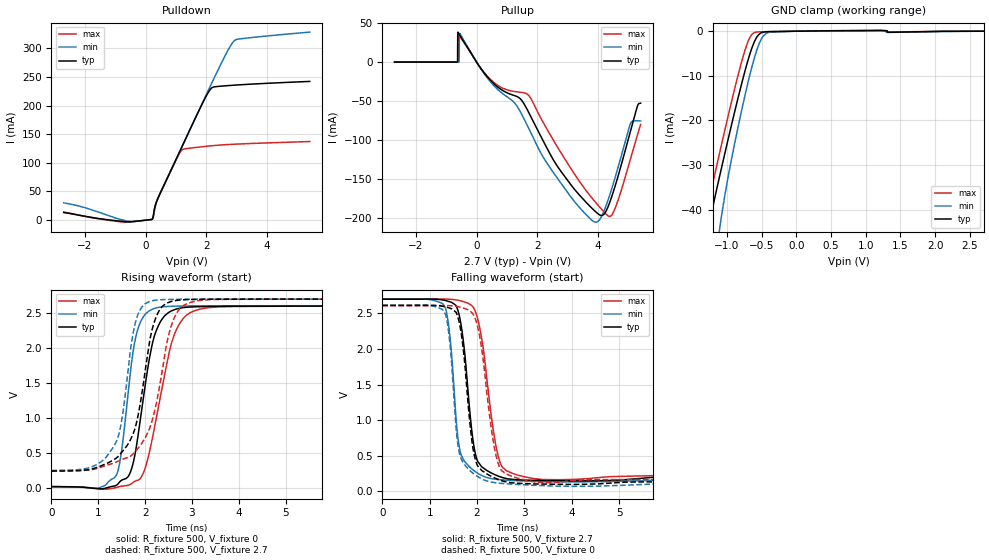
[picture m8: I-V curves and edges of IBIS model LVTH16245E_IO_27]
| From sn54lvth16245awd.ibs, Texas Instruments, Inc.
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[Model]   LVTH16245E_IO_27
Model_type  I/O
Vinl=0.945
Vinh=1.75
Enable   Active-Low
Vref =   0
Rref =   500
Cref =   50p
Vmeas =   1.5
| variable   typ   min   max
C_comp   3.31pF   2.51pF   4.02pF
| C_pullup   5.53pF   0.96pF   13.97pF
| C_pulldown   3.35pF   2.55pF   4.14pF
| C_tri-state   3.31pF   2.51pF   4.02pF
[Temperature Range]   40   100   -40
| Ambient temperature   25   85   -40
[Voltage range]   2.7   2.7   2.7
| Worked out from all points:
|   slope of the pulldown table from 0 to 0.405 V, typ, clamps not added: 10.5 ohm
|   slope of the pullup table from 0 to 0.405 V, typ, clamps not added: 19.2 ohm
|   GND clamp passes 1 mA (typ) near -0.55 V on its own axis
|   rising waveform, R_fixture 500, V_fixture 0: 20-80 % time 364ps typ, 280ps min, 471ps max; typ from 0.015 V to 2.6 V
|   falling waveform, R_fixture 500, V_fixture 2.7: 20-80 % time 223ps typ, 181ps min, 292ps max; typ from 2.7 V to 0.214 V
|   rising waveform, R_fixture 500, V_fixture 2.7: 20-80 % time 412ps typ, 317ps min, 496ps max; typ from 0.238 V to 2.7 V
|   falling waveform, R_fixture 500, V_fixture 0: 20-80 % time 233ps typ, 200ps min, 299ps max; typ from 2.61 V to 0.055 V
[GND Clamp]
| LVTH16245E_IO_27
|   Voltage   I(typ)   I(min)   I(max)
-2.7V     -481.8mA   -527.9mA   -418.4mA
-1.35V    -52.43mA   -85.91mA   -44.38mA
-1.325V   -49.75mA   -80mA      -42.6mA
-1.26V    -43.79mA   -66.47mA   -38mA
-1.09V    -31.44mA   -42.64mA   -26.22mA
-950mV    -22.04mA   -29.94mA   -16.83mA
-780mV    -11.26mA   -17.15mA   -6.356mA
-695mV    -6.416mA   -11.38mA   -2.245mA
-605mV    -2.337mA   -5.992mA   -317uA
-505mV    -358.1uA   -1.752mA   -132.5uA
-390mV    -91.77uA   -205.4uA   -101uA
2.7V      154.1pA    18.32nA    25.91pA
[Pulldown]
| LVTH16245E_IO_27
|   Voltage   I(typ)   I(min)   I(max)
-2.7V     13.23mA    30.13mA    14.3mA
-630mV    -2.788mA   -1.362mA   -3.609mA
215mV     1.883mA    1.702mA    1.527mA
250mV     8.001mA    5.839mA    6.518mA
320mV     26.43mA    26.38mA    25.33mA
410mV     39.07mA    38.84mA    39.68mA
1.19V     127.9mA    127.5mA    122.4mA
1.865V    203.5mA    204.5mA    128.1mA
2.135V    228.8mA    234.9mA    129.6mA
2.88V     235.4mA    311.1mA    132.4mA
3.1V      236.2mA    316.4mA    132.9mA
5.4V      242.1mA    328.2mA    137.2mA
[Pullup]
| LVTH16245E_IO_27
|   Voltage   I(typ)   I(min)   I(max)
-2.7V     48.42uA    63.67uA    38.84uA
-630mV    35.26uA    49.1uA     35.52uA
-620mV    37.07mA    47.29uA    33.5uA
-585mV    36.43mA    55.2uA     34.43mA
-550mV    34.18mA    36.72mA    32.63mA
545mV     -26.71mA   -29.04mA   -25.28mA
1.725V    -65.07mA   -85.36mA   -43.03mA
3.23V     -163.1mA   -178.7mA   -143.6mA
4.1V      -196.2mA   -198.3mA   -187.5mA
4.515V    -164.3mA   -153.5mA   -191.2mA
5.065V    -88.53mA   -78.66mA   -124mA
5.4V      -52.53mA   -75.34mA   -79.73mA
[Ramp]
| LVTH16245E_IO_27
| variable   typ   min   max
dV/dt_r   1.57/3.70E-10   1.57/2.86E-10   1.57/4.86E-10
dV/dt_f   1.53/2.38E-10   1.54/1.96E-10   1.52/3.09E-10
R_load = 500
[Rising Waveform]
| LVTH16245E_IO_27
R_fixture =   500
C_fixture =   0
L_fixture =   0
V_fixture =   0
V_fixture_min = 0
V_fixture_max = 0
|   Time   V(typ)   V(min)   V(max)
0s        14.77mV    17mV       12.18mV
1.355ns   24.71mV    149.8mV    -2.295mV
1.475ns   93.79mV    417.5mV    18.02mV
1.645ns   164.8mV    1.392V     35.54mV
1.88ns    885.4mV    2.335V     118.9mV
2.12ns    1.944V     2.543V     590.5mV
2.315ns   2.36V      2.584V     1.26V
2.705ns   2.564V     2.599V     2.309V
3.4ns     2.594V     2.603V     2.58V
24.25ns   2.6V       2.605V     2.599V
[Falling Waveform]
| LVTH16245E_IO_27
R_fixture =   500
C_fixture =   0
L_fixture =   0
V_fixture =   2.7
V_fixture_min = 2.7
V_fixture_max = 2.7
|   Time   V(typ)   V(min)   V(max)
0s        2.7V       2.7V       2.7V
1.31ns    2.684V     2.604V     2.702V
1.43ns    2.662V     2.163V     2.699V
1.56ns    2.607V     992mV      2.69V
1.665ns   2.331V     508.5mV    2.675V
1.965ns   524.8mV    274.1mV    2.526V
2.35ns    240.2mV    171.2mV    827.2mV
2.545ns   190.2mV    158.4mV    330.4mV
3.425ns   149.7mV    133.8mV    163.7mV
24.25ns   214.2mV    209.1mV    236.9mV
[Rising Waveform]
| LVTH16245E_IO_27
R_fixture =   500
C_fixture =   0
L_fixture =   0
V_fixture =   2.7
V_fixture_min = 2.7
V_fixture_max = 2.7
|   Time   V(typ)   V(min)   V(max)
0s        237.6mV    245.6mV    242.1mV
1.17ns    342.7mV    436.5mV    318.5mV
1.44ns    456.3mV    763.3mV    383.9mV
1.63ns    616.8mV    1.635V     431.5mV
1.835ns   982.2mV    2.456V     552.5mV
2.1ns     2.105V     2.666V     855.6mV
2.22ns    2.414V     2.684V     1.144V
2.615ns   2.674V     2.695V     2.418V
3.215ns   2.696V     2.699V     2.684V
24.25ns   2.7V       2.7V       2.7V
[Falling Waveform]
| LVTH16245E_IO_27
R_fixture =   500
C_fixture =   0
L_fixture =   0
V_fixture =   0
V_fixture_min = 0
V_fixture_max = 0
|   Time   V(typ)   V(min)   V(max)
0s        2.611V     2.616V     2.609V
1.31ns    2.596V     2.517V     2.611V
1.425ns   2.575V     2.09V      2.609V
1.56ns    2.513V     869.5mV    2.599V
1.69ns    2.104V     421mV      2.579V
1.94ns    511mV      239.7mV    2.462V
2.345ns   195mV      122.6mV    691.7mV
2.53ns    145.4mV    108.7mV    280.3mV
3.375ns   100.3mV    78.28mV    121.6mV
24.25ns   55.04mV    28.49mV    82.34mV
